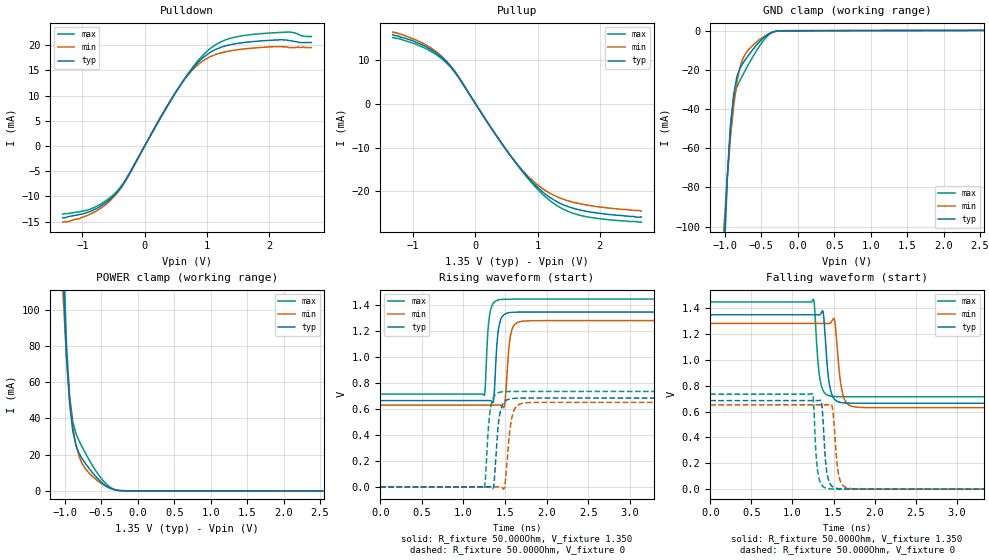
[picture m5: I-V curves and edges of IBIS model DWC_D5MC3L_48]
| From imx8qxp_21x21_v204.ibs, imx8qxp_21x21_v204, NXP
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[Model] DWC_D5MC3L_48
Model_type   I/O
Polarity   Non-Inverting
Enable   Active-High
C_comp   1.262pF   1.180pF   1.365pF
C_comp_pullup   279.441fF   258.852fF   306.885fF
C_comp_pulldown 973.651fF   908.565fF   1.053pF
Vinh = 800.000mV
Vinl = 550.000mV
Vmeas = 675.000mV
Vref = 675.000mV
Rref = 50Ohms
Cref = 0pF
[Model Spec]
Vinh   800.000mV   766.500mV   850.000mV
Vinl   550.000mV   516.500mV   600.000mV
Vmeas   675.000mV   641.500mV   725.000mV
Vref   675.000mV   641.500mV   725.000mV
D_overshoot_ampl_h 0.4 NA   NA
D_overshoot_ampl_l 0.4 NA   NA
D_overshoot_area_l 100.000p NA   NA
D_overshoot_area_h 100.000p NA   NA
[Receiver Thresholds]
Vth = 675.000mV
Vth_min = 661.500mV
Vth_max = 688.500mV
Vinh_ac = 125.000mV
Vinh_dc = 90.000mV
Vinl_ac = -125.000mV
Vinl_dc = -90.000mV
Tslew_ac = 5.000ns
Threshold_sensitivity = 0.5
Reference_supply Pullup_ref
[Temperature Range]   25.000   125.000   -40.000
[Voltage Range]   1.350V   1.283V   1.450V
[GND Clamp Reference]   0.00V   0.00V   0.00V
|[C Comp Corner]
| variable   typ   min   max
|C_comp 1.262pF   1.365pF   1.180pF
|C_comp_pullup 279.441fF   306.885fF   258.852fF
|C_comp_pulldown 973.651fF   1.053pF   908.565fF
[Pulldown Reference]   0.00V   0.00V   0.00V
[POWER Clamp Reference]   1.350V   1.283V   1.450V
[Pullup Reference]   1.350V   1.283V   1.450V
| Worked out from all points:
|   slope of the pulldown table from 0 to 0.203 V, typ, clamps not added: 45.3 ohm
|   slope of the pullup table from 0 to 0.203 V, typ, clamps not added: 45.8 ohm
|   GND clamp passes 1 mA (typ) near -0.36 V on its own axis
|   POWER clamp passes 1 mA (typ) near -0.36 V on its own axis
|   rising waveform, R_fixture 50.000Ohm, V_fixture 1.350: 20-80 % time 43.3ps typ, 48.8ps min, 40.9ps max; typ from 0.665 V to 1.35 V
|   rising waveform, R_fixture 50.000Ohm, V_fixture 0: 20-80 % time 53.2ps typ, 61.6ps min, 49.3ps max; typ from 0 V to 0.685 V
|   falling waveform, R_fixture 50.000Ohm, V_fixture 1.350: 20-80 % time 57.5ps typ, 65.2ps min, 53.3ps max; typ from 1.35 V to 0.665 V
|   falling waveform, R_fixture 50.000Ohm, V_fixture 0: 20-80 % time 46.2ps typ, 53ps min, 41.5ps max; typ from 0.685 V to 0 V
[GND Clamp]
-1.318V   -593.4mA   -427mA     -758.7mA
-1.011V   -108.7mA   -99.8mA    -118.2mA
-966.7mV  -74.7mA    -74.6mA    -75.87mA
-922.7mV  -49.41mA   -54.3mA    -47.9mA
-878.8mV  -32.42mA   -38.21mA   -34.12mA
-834.8mV  -23.33mA   -26.23mA   -28.72mA
-790.9mV  -19.01mA   -18.35mA   -25.26mA
-747mV    -16.25mA   -13.76mA   -22.11mA
-483.3mV  -4.093mA   -3.434mA   -5.633mA
-351.5mV  -766.8uA   -911.3uA   -894.7uA
-263.6mV  -79.41uA   -192.1uA   -51.43uA
2.68V     154.9uA    127.3uA    193.1uA
[Power Clamp]
-1.33V    727.8mA    510.6mA    954.1mA
-1.023V   119.4mA    107.4mA    137.5mA
-978.8mV  74.87mA    74.2mA     82.23mA
-934.8mV  47.95mA    50.66mA    52.21mA
-890.9mV  32.9mA     35.12mA    38.1mA
-847mV    24.9mA     25.11mA    31.53mA
-759.1mV  17.5mA     14.71mA    23.9mA
-671.2mV  12.54mA    9.915mA    17.38mA
-495.5mV  4.603mA    3.922mA    6.563mA
-363.6mV  1.088mA    1.21mA     1.541mA
-231.8mV  46.56uA    141.4uA    53.69uA
2.668V    -76.24uA   -66.58uA   -87.76uA
[Pulldown]
-1.318V   -14.2mA    -15.1mA    -13.5mA
-834.8mV  -12.76mA   -13.26mA   -12.32mA
-615.2mV  -11.12mA   -11.48mA   -10.77mA
-439.4mV  -9.099mA   -9.296mA   -8.898mA
-307.6mV  -6.807mA   -6.963mA   -6.694mA
483.3mV   10.32mA    10.4mA     10.28mA
703mV     14.3mA     14.14mA    14.42mA
922.7mV   17.33mA    16.73mA    17.81mA
1.186V    19.37mA    18.31mA    20.39mA
1.538V    20.41mA    19.15mA    21.77mA
2.329V    20.88mA    19.5mA     22.57mA
2.68V     20.5mA     19.5mA     21.7mA
[Pullup]
-1.33V    15.7mA     16.3mA     15.06mA
-803mV    13.01mA    13.43mA    12.56mA
-627.3mV  11.5mA     11.8mA     11.12mA
-451.5mV  9.33mA     9.507mA    9.082mA
-275.8mV  6.124mA    6.257mA    6.022mA
207.6mV   -4.531mA   -4.616mA   -4.5mA
559.1mV   -11.74mA   -11.76mA   -11.77mA
822.7mV   -16.45mA   -16.18mA   -16.66mA
1.086V    -20.16mA   -19.42mA   -20.71mA
1.35V     -22.61mA   -21.44mA   -23.56mA
1.658V    -24.15mA   -22.73mA   -25.34mA
2.668V    -25.8mA    -24.45mA   -27mA
[Ramp]
R_load=50.000Ohm
dV/dt_r   410.400mV/49.000ps  390.957mV/55.500ps  440.100mV/45.000ps
dV/dt_f   410.370mV/52.000ps  390.927mV/59.500ps  440.070mV/48.500ps
[Rising waveform]
R_fixture=50.000Ohm
V_fixture=1.350
V_fixture_min=1.283
V_fixture_max=1.450
0s        665mV      630.5mV    715.6mV
1.253ns   665mV      630.5mV    705.4mV
1.323ns   665.9mV    630.6mV    1.355V
1.363ns   666.2mV    630.5mV    1.42V
1.413ns   1.175V     631.4mV    1.44V
1.464ns   1.311V     623.1mV    1.446V
1.494ns   1.331V     626.2mV    1.447V
1.574ns   1.345V     1.192V     1.447V
1.704ns   1.348V     1.277V     1.448V
10ns      1.348V     1.282V     1.448V
[Rising waveform]
R_fixture=50.000Ohm
V_fixture=0
0s        428.7nV    9.028uV    56.87nV
1.253ns   8.208uV    7.839uV    -11.49mV
1.333ns   278.6uV    15.22uV    632mV
1.363ns   -1.975mV   -71.11uV   691.3mV
1.423ns   501.2mV    1.061mV    726.7mV
1.474ns   638.2mV    -10.53mV   733.4mV
1.504ns   662.4mV    42.65mV    734.7mV
1.584ns   681.2mV    541.4mV    735.8mV
1.744ns   685.1mV    647.9mV    735.9mV
10ns      684.8mV    652.1mV    735.1mV
[Falling waveform]
R_fixture=50.000Ohm
V_fixture=1.350
V_fixture_min=1.283
V_fixture_max=1.450
0s        1.348V     1.282V     1.448V
1.253ns   1.348V     1.282V     1.47V
1.343ns   1.354V     1.282V     823.3mV
1.373ns   1.375V     1.282V     762.8mV
1.434ns   882.4mV    1.281V     724.7mV
1.484ns   724.8mV    1.304V     717.5mV
1.514ns   693.9mV    1.305V     715.9mV
1.614ns   667.9mV    730.4mV    714.6mV
1.774ns   664.5mV    634.7mV    714.5mV
10ns      664.9mV    630.5mV    715.4mV
[Falling waveform]
R_fixture=50.000Ohm
V_fixture=0
0s        684.6mV    652mV      734.8mV
1.243ns   684.6mV    652mV      739.3mV
1.313ns   684.3mV    652mV      113.5mV
1.353ns   678mV      652.1mV    34.42mV
1.403ns   213.2mV    651.7mV    9.006mV
1.444ns   61.39mV    653.5mV    3.183mV
1.484ns   21.75mV    637mV      1.18mV
1.574ns   3.085mV    79.66mV    133.7uV
1.714ns   196.3uV    4.291mV    11.41uV
10ns      675.5nV    9.3uV      117.7nV
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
